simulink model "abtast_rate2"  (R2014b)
settings: Solver=FixedStepDiscrete  StartTime=0.0  StopTime=0.05  RelTol=1e-3
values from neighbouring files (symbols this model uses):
  ampl = 1    [abtast_rate_1.m]    (also in ad_test_12.m; ad_test_2.m; ad_test_3.m; fft_1.m = 10)
  fsig = 100    [abtast_rate_1.m]    (also in ad_test_12.m = ',num2str(fsig),'; ad_test_2.m = ',num2str(fsig),'; ad_test_3.m = ',num2str(fsig),'; leakage_2.m = 100.5)
  Ts = 1/fs    (= 0.00025)    [abtast_rate_1.m]    (also in ad_test_12.m = 0.0009765625; ad_test_2.m = 0.00048828125; ad_test_3.m = 0.00048828125; DA_wandler_spektr_1.m = 0.01)
  Ts1 = 1/1000    (= 0.001)    [abtast_rate_1.m]
  Ts2 = Ts1/4    (= 0.00025)    [abtast_rate_1.m]

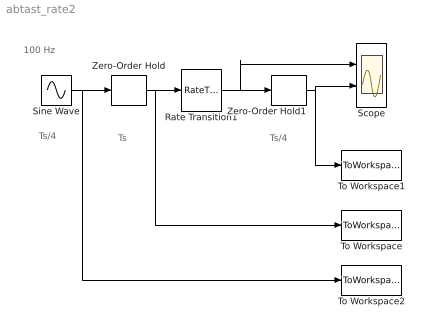
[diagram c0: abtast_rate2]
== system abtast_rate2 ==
  note: Ts/4
  note: 100 Hz
  note: Ts/4
  note: Ts
  Rate Transition1 : RateTransition  OutPortSampleTimeOpt=Inherit  OutPortSampleTime=1/4000
  Scope : Scope  NumInputPorts=2
  Sine Wave : Sin  Amplitude=ampl  Frequency=2*pi*fsig  SampleTime=Ts
  To Workspace : ToWorkspace  VariableName=y1  SaveFormat=Timeseries  SampleTime=-1
  To Workspace1 : ToWorkspace  VariableName=y2  SaveFormat=Timeseries  SampleTime=-1
  To Workspace2 : ToWorkspace  VariableName=y  SaveFormat=Timeseries  SampleTime=-1
  Zero-Order Hold : ZeroOrderHold  SampleTime=Ts1
  Zero-Order Hold1 : ZeroOrderHold  SampleTime=Ts2
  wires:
  Sine Wave/1 -> To Workspace2/1, Zero-Order Hold/1
  Zero-Order Hold1/1 -> To Workspace1/1, Scope/2
  Zero-Order Hold/1 -> To Workspace/1, Rate Transition1/1
  Rate Transition1/1 -> Scope/1, Zero-Order Hold1/1
